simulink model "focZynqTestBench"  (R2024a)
settings: Solver=VariableStepAuto  StartTime=0.0  StopTime=8  RelTol=1e-3
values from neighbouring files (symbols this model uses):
  inverter = Avnet Zynq AD-FMCMOTCON2
                24.0
                5.0
                1
                0    [focZynqData.sldd]
  sampleTime = 4.0E-5
                0.001
                0.001
                4.0E-5
                2.0E-8
                4.0E-5
                0.001
                2.0E-8
                2.0E-8
                2.0E-8    [focZynqData.sldd]
libraries: motorAndLoadSimPowerSystemsLib x1, SignalEditorBlockLib x1

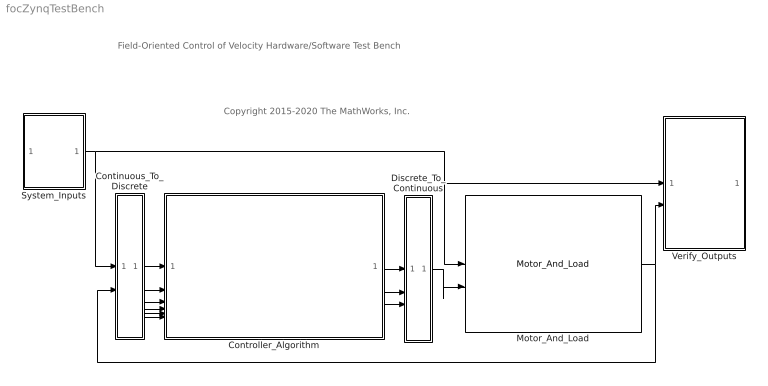
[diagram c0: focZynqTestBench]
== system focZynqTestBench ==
  note: Field-Oriented Control of Velocity Hardware/Software Test Bench
  note: Copyright 2015-2020 The MathWorks, Inc.
  Continuous_To_Discrete : Subsystem
  Controller_Algorithm : Subsystem  DataTypeOverrideAppliesTo=Fixed-point
  Discrete_To_Continuous : Subsystem  Description=""
  Motor_And_Load : motorAndLoadSimPowerSystemsLib/Motor_And_Load  SystemSampleTime=-1  VariantActivationTime=update diagram  AllowFlexibleInterface=on  Latency=0  AutoFrameSizeCalculation=off
  System_Inputs : Subsystem  Description=""
  Verify_Outputs : Subsystem  Description=|
      | System Analysis for Speed Control Design
      | 
      | Analyize and plot signals used to analyize performance of
      | speed  control designs
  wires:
  Discrete_To_Continuous/1(Motor_Commands) -> Motor_And_Load/2
  Motor_And_Load/1 -> Verify_Outputs/2(System_Measurements), Continuous_To_Discrete/2(Motor_Measurements)
  System_Inputs/1(System_Inputs) -> Continuous_To_Discrete/1(System_Inputs), Motor_And_Load/1, Verify_Outputs/1(System_Inputs)
  Continuous_To_Discrete/1(Motor_On) -> Controller_Algorithm/1(Motor_On)
  Continuous_To_Discrete/2(Command_Type) -> Controller_Algorithm/2(Command_Type)
  Continuous_To_Discrete/3(Velocity_Command) -> Controller_Algorithm/3(Velocity_Command)
  Continuous_To_Discrete/4(ADC_Count) -> Controller_Algorithm/4(ADC_Count)
  Continuous_To_Discrete/5(Encoder_Index_Found) -> Controller_Algorithm/5(Encoder_Index_Found)
  Continuous_To_Discrete/6(Encoder_Count) -> Controller_Algorithm/6(Encoder_Count)
  Controller_Algorithm/1(Controller_Mode) -> Discrete_To_Continuous/1(Controller_Mode)
  Controller_Algorithm/2(Inverter_Enable) -> Discrete_To_Continuous/2(Inverter_Enable)
  Controller_Algorithm/3(PWM_Compare) -> Discrete_To_Continuous/3(PWM_Compare)

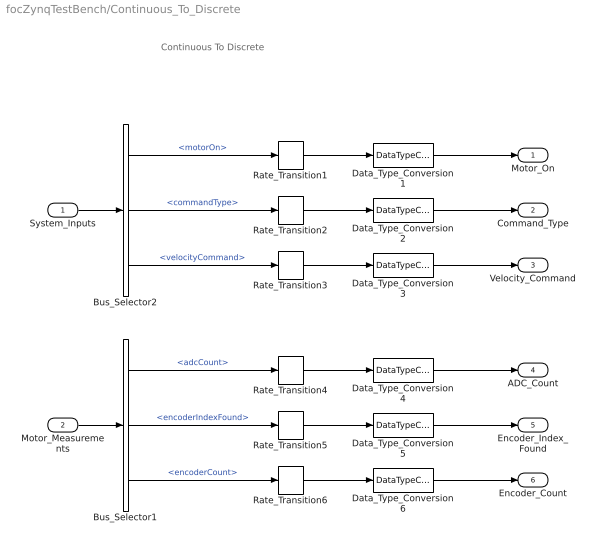
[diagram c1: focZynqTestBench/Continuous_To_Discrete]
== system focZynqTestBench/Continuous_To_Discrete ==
  note: Continuous To Discrete
  System_Inputs : Inport
  Motor_Measurements : Inport  Port=2
  Bus_Selector1 : BusSelector  OutputSignals=adcCount,encoderIndexFound,encoderCount
  Bus_Selector2 : BusSelector  OutputSignals=motorOn,commandType,velocityCommand
  Data_Type_Conversion{1..6} (6 alike) : DataTypeConversion
  Rate_Transition{1..6} (6 alike) : RateTransition  Integrity=off  Deterministic=off
  Motor_On : Outport
  Command_Type : Outport  Port=2
  Velocity_Command : Outport  Port=3
  ADC_Count : Outport  Port=4
  Encoder_Index_Found : Outport  Port=5
  Encoder_Count : Outport  Port=6
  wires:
  Bus_Selector2/3 -> Rate_Transition3/1  "<velocityCommand>"
  Bus_Selector2/2 -> Rate_Transition2/1  "<commandType>"
  Bus_Selector2/1 -> Rate_Transition1/1  "<motorOn>"
  System_Inputs/1 -> Bus_Selector2/1
  Bus_Selector1/3 -> Rate_Transition6/1  "<encoderCount>"
  Bus_Selector1/2 -> Rate_Transition5/1  "<encoderIndexFound>"
  Bus_Selector1/1 -> Rate_Transition4/1  "<adcCount>"
  Data_Type_Conversion6/1 -> Encoder_Count/1
  Data_Type_Conversion5/1 -> Encoder_Index_Found/1
  Rate_Transition6/1 -> Data_Type_Conversion6/1
  Rate_Transition5/1 -> Data_Type_Conversion5/1
  Rate_Transition1/1 -> Data_Type_Conversion1/1
  Data_Type_Conversion1/1 -> Motor_On/1
  Motor_Measurements/1 -> Bus_Selector1/1
  Data_Type_Conversion4/1 -> ADC_Count/1
  Rate_Transition4/1 -> Data_Type_Conversion4/1
  Rate_Transition3/1 -> Data_Type_Conversion3/1
  Data_Type_Conversion3/1 -> Velocity_Command/1
  Data_Type_Conversion2/1 -> Command_Type/1
  Rate_Transition2/1 -> Data_Type_Conversion2/1

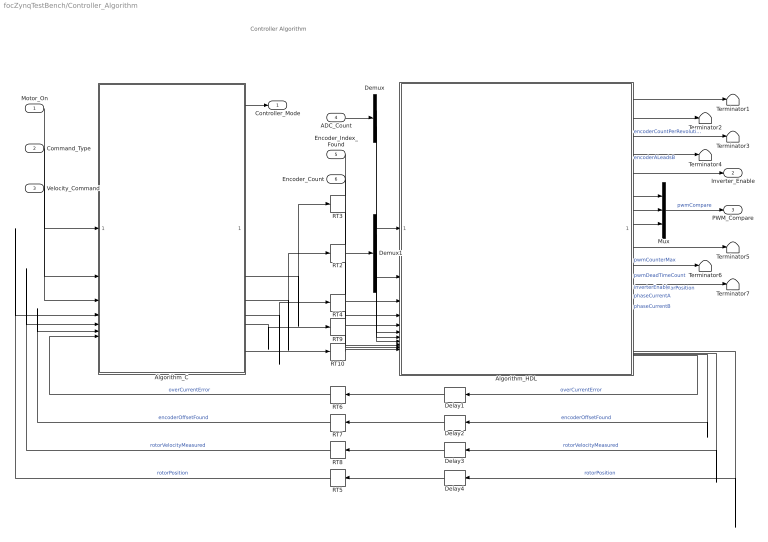
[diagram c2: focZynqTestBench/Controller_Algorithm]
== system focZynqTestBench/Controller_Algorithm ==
  note: Controller Algorithm
  Motor_On : Inport  SampleTime=sampleTime.VelocityControl  Interpolate=off
  Command_Type : Inport  Port=2  Interpolate=off
  Velocity_Command : Inport  Port=3
  ADC_Count : Inport  Port=4  PortDimensions=2  SampleTime=sampleTime.CurrentControl  Interpolate=off
  Encoder_Index_Found : Inport  Port=5  Interpolate=off
  Encoder_Count : Inport  Port=6  Interpolate=off
  Algorithm_C : ModelReference  ModelNameDialog=focZynqC  SimulationMode=Normal  ModelReferenceVersion=8.2
  Algorithm_HDL : ModelReference  ModelNameDialog=focZynqHdl  SimulationMode=Normal  ModelReferenceVersion=8.1
  Delay{1..4} (4 alike) : Delay  DelayLength=1
  Demux : Demux  Outputs=2
  Demux1 : Demux  Outputs=3
  Mux : Mux  Inputs=3
  RT{2..10} (9 alike) : RateTransition  Integrity=off
  Terminator{1..7} (7 alike) : Terminator
  Controller_Mode : Outport
  Inverter_Enable : Outport  Port=2
  PWM_Compare : Outport  Port=3
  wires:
  Algorithm_HDL/4 -> Terminator4/1  "pwmDeadTimeCount"
  Algorithm_HDL/11 -> Terminator7/1  "rotorPosition"
  Algorithm_HDL/3 -> Terminator3/1  "pwmCounterMax"
  Demux1/3 -> Algorithm_HDL/8
  Demux1/2 -> Algorithm_HDL/7
  Demux1/1 -> Algorithm_HDL/6
  RT10/1 -> Algorithm_HDL/11
  RT9/1 -> Algorithm_HDL/10
  RT4/1 -> Algorithm_HDL/9
  Algorithm_C/4 -> RT4/1
  Algorithm_C/5 -> RT9/1
  Algorithm_C/6 -> RT10/1
  Algorithm_HDL/10 -> Terminator6/1  "phaseCurrentB"
  Algorithm_HDL/8 -> Mux/3
  Algorithm_HDL/7 -> Mux/2
  Algorithm_HDL/6 -> Mux/1
  ADC_Count/1 -> Demux/1
  Demux/2 -> Algorithm_HDL/2
  Demux/1 -> Algorithm_HDL/1
  Algorithm_HDL/2 -> Terminator2/1  "encoderALeadsB"
  Algorithm_HDL/1 -> Terminator1/1  "encoderCountPerRevolution"
  Algorithm_HDL/13 -> Delay3/1  "rotorVelocityMeasured"
  Delay3/1 -> RT8/1
  RT8/1 -> Algorithm_C/5  "rotorVelocityMeasured"
  Algorithm_C/1 -> Controller_Mode/1
  Algorithm_C/2 -> RT3/1
  Algorithm_C/3 -> RT2/1
  Encoder_Index_Found/1 -> Algorithm_HDL/3
  Encoder_Count/1 -> Algorithm_HDL/4
  Algorithm_HDL/9 -> Terminator5/1  "phaseCurrentA"
  RT7/1 -> Algorithm_C/6  "encoderOffsetFound"
  RT6/1 -> Algorithm_C/7  "overCurrentError"
  RT5/1 -> Algorithm_C/4  "rotorPosition"
  Mux/1 -> PWM_Compare/1  "pwmCompare"
  Algorithm_HDL/14 -> Delay2/1  "encoderOffsetFound"
  Delay4/1 -> RT5/1
  Delay1/1 -> RT6/1
  Delay2/1 -> RT7/1
  Command_Type/1 -> Algorithm_C/2
  Motor_On/1 -> Algorithm_C/1
  Velocity_Command/1 -> Algorithm_C/3
  RT2/1 -> Demux1/1
  RT3/1 -> Algorithm_HDL/5
  Algorithm_HDL/15 -> Delay1/1  "overCurrentError"
  Algorithm_HDL/12 -> Delay4/1  "rotorPosition"
  Algorithm_HDL/5 -> Inverter_Enable/1  "inverterEnable"

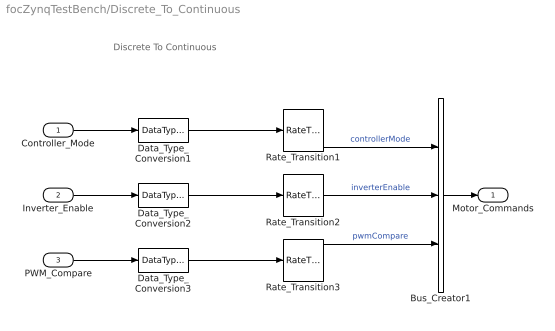
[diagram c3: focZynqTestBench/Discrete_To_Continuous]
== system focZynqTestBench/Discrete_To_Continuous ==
  note: Discrete To Continuous
  Controller_Mode : Inport
  Inverter_Enable : Inport  Port=2
  PWM_Compare : Inport  Port=3
  Bus_Creator1 : BusCreator  Inputs=3
  Data_Type_Conversion1 : DataTypeConversion  OutDataTypeStr=Enum: modeSchedulerEnum
  Data_Type_Conversion2 : DataTypeConversion
  Data_Type_Conversion3 : DataTypeConversion
  Rate_Transition1 : RateTransition  Integrity=off  Deterministic=off
  Rate_Transition2 : RateTransition  Integrity=off  Deterministic=off
  Rate_Transition3 : RateTransition  Integrity=off  Deterministic=off
  Motor_Commands : Outport
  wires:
  Controller_Mode/1 -> Data_Type_Conversion1/1
  Data_Type_Conversion1/1 -> Rate_Transition1/1
  Rate_Transition3/1 -> Bus_Creator1/3  "pwmCompare"
  Rate_Transition2/1 -> Bus_Creator1/2  "inverterEnable"
  PWM_Compare/1 -> Data_Type_Conversion3/1
  Data_Type_Conversion3/1 -> Rate_Transition3/1
  Inverter_Enable/1 -> Data_Type_Conversion2/1
  Data_Type_Conversion2/1 -> Rate_Transition2/1
  Bus_Creator1/1 -> Motor_Commands/1
  Rate_Transition1/1 -> Bus_Creator1/1  "controllerMode"

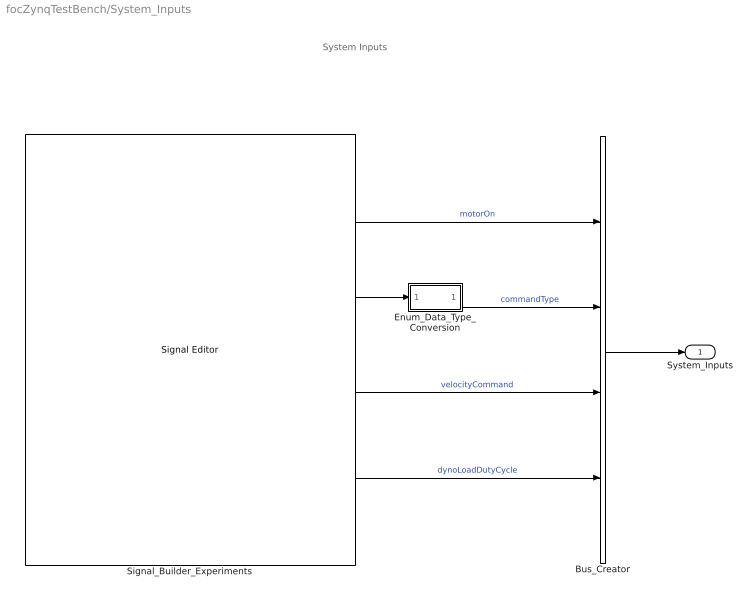
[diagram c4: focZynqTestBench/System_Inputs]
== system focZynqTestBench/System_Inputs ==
  note: System Inputs
  Bus_Creator : BusCreator  Inputs=4
  Enum_Data_Type_Conversion : Subsystem  mask(Convert to enumerated data type){dataTypeStr=Enum: commandTypeEnum}
      mask prompts: dataTypeStr "Output data type"
  Signal_Builder_Experiments : SignalEditorBlockLib/Signal Editor  FileName=TestBenchInputs.mat  ActiveScenario=Closed_loop_velocity_steps  ActiveSignal=dynoLoadDutyCycle (Percent)  IsBus=off  OutputBusObjectStr=Bus: BusObject  SampleTime=-1  ZeroCross=off  OutputAfterFinalValue=Extrapolation  Unit=inherit  PreserveSignalName=on  ApplySigPropsToAllScenarios=on  ApplySigPropsToAllSignals=off
  System_Inputs : Outport
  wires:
  Bus_Creator/1 -> System_Inputs/1
  Enum_Data_Type_Conversion/1(Out) -> Bus_Creator/2  "commandType"
  Signal_Builder_Experiments/4 -> Bus_Creator/4  "dynoLoadDutyCycle"
  Signal_Builder_Experiments/3 -> Bus_Creator/3  "velocityCommand"
  Signal_Builder_Experiments/2 -> Enum_Data_Type_Conversion/1(In)
  Signal_Builder_Experiments/1 -> Bus_Creator/1  "motorOn"

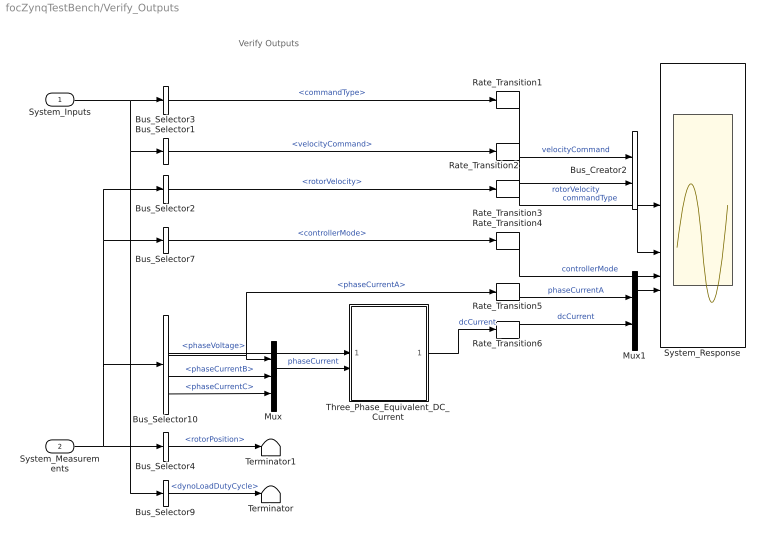
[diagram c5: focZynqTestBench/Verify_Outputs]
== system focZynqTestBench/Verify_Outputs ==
  note: Verify Outputs
  System_Inputs : Inport
  System_Measurements : Inport  Port=2
  Bus_Creator2 : BusCreator  Inputs=2
  Bus_Selector1 : BusSelector  OutputSignals=velocityCommand
  Bus_Selector10 : BusSelector  OutputSignals=phaseVoltage,motor.phaseCurrentA,motor.phaseCurrentB,motor.phaseCurrentC
  Bus_Selector2 : BusSelector  OutputSignals=motor.rotorVelocity
  Bus_Selector3 : BusSelector  OutputSignals=commandType
  Bus_Selector4 : BusSelector  OutputSignals=motor.rotorPosition
  Bus_Selector7 : BusSelector  OutputSignals=controller.controllerMode
  Bus_Selector9 : BusSelector  OutputSignals=dynoLoadDutyCycle
  Mux : Mux  Inputs=3
  Mux1 : Mux  Inputs=2
  Rate_Transition{1..6} (6 alike) : RateTransition  Integrity=off
  System_Response : Scope  NumInputPorts=4
  Terminator : Terminator
  Terminator1 : Terminator
  Three_Phase_Equivalent_DC_Current : Subsystem
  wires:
  Bus_Selector4/1 -> Terminator1/1  "<rotorPosition>"
  Bus_Selector3/1 -> Rate_Transition1/1  "<commandType>"
  Mux/1 -> Three_Phase_Equivalent_DC_Current/2(Iabc)  "phaseCurrent"
  Bus_Selector7/1 -> Rate_Transition4/1  "<controllerMode>"
  Bus_Selector1/1 -> Rate_Transition2/1  "<velocityCommand>"
  Bus_Selector2/1 -> Rate_Transition3/1  "<rotorVelocity>"
  Bus_Selector9/1 -> Terminator/1  "<dynoLoadDutyCycle>"
  Bus_Selector10/2 -> Mux/1, Rate_Transition5/1  "<phaseCurrentA>"
  Bus_Selector10/3 -> Mux/2  "<phaseCurrentB>"
  Bus_Selector10/4 -> Mux/3  "<phaseCurrentC>"
  Bus_Selector10/1 -> Three_Phase_Equivalent_DC_Current/1(Vabc)  "<phaseVoltage>"
  Three_Phase_Equivalent_DC_Current/1(Idc) -> Rate_Transition6/1  "dcCurrent"
  Mux1/1 -> System_Response/4
  Rate_Transition4/1 -> System_Response/3  "controllerMode"
  Bus_Creator2/1 -> System_Response/2
  Rate_Transition1/1 -> System_Response/1  "commandType"
  System_Inputs/1 -> Bus_Selector1/1, Bus_Selector9/1, Bus_Selector3/1
  System_Measurements/1 -> Bus_Selector2/1, Bus_Selector7/1, Bus_Selector10/1, Bus_Selector4/1
  Rate_Transition2/1 -> Bus_Creator2/1  "velocityCommand"
  Rate_Transition3/1 -> Bus_Creator2/2  "rotorVelocity"
  Rate_Transition5/1 -> Mux1/1  "phaseCurrentA"
  Rate_Transition6/1 -> Mux1/2  "dcCurrent"

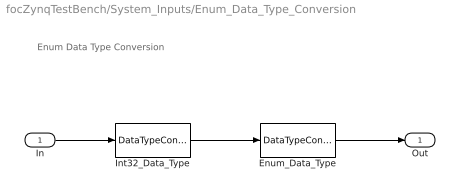
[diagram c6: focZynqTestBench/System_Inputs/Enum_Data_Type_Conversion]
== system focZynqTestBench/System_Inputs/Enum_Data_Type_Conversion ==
  note: Enum Data Type Conversion
  In : Inport
  Enum_Data_Type : DataTypeConversion  OutDataTypeStr=dataTypeStr
  Int32_Data_Type : DataTypeConversion  OutDataTypeStr=int32
  Out : Outport
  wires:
  In/1 -> Int32_Data_Type/1
  Int32_Data_Type/1 -> Enum_Data_Type/1
  Enum_Data_Type/1 -> Out/1

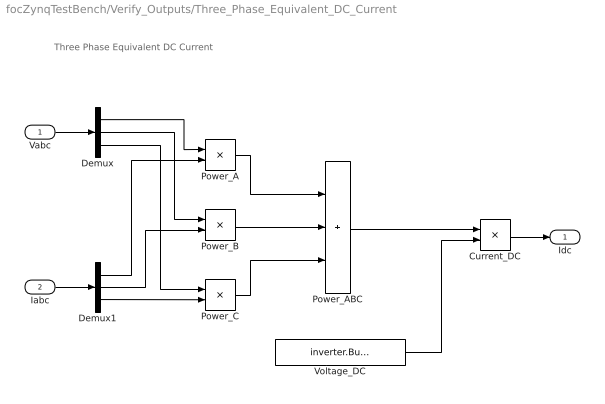
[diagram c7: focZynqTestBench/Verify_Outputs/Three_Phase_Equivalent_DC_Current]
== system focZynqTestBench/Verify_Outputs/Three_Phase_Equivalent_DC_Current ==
  note: Three Phase Equivalent DC Current
  Vabc : Inport
  Iabc : Inport  Port=2
  Current_DC : Product  Inputs=*/
  Demux : Demux  Outputs=3
  Demux1 : Demux  Outputs=3
  Power_A : Product
  Power_ABC : Sum  Inputs=+++
  Power_B : Product
  Power_C : Product
  Voltage_DC : Constant  Value=inverter.BusVoltage
  Idc : Outport
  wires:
  Demux/3 -> Power_C/1
  Demux/2 -> Power_B/1
  Demux/1 -> Power_A/1
  Power_ABC/1 -> Current_DC/1
  Voltage_DC/1 -> Current_DC/2
  Current_DC/1 -> Idc/1
  Power_C/1 -> Power_ABC/3
  Vabc/1 -> Demux/1
  Power_B/1 -> Power_ABC/2
  Power_A/1 -> Power_ABC/1
  Demux1/1 -> Power_A/2
  Demux1/2 -> Power_B/2
  Demux1/3 -> Power_C/2
  Iabc/1 -> Demux1/1
